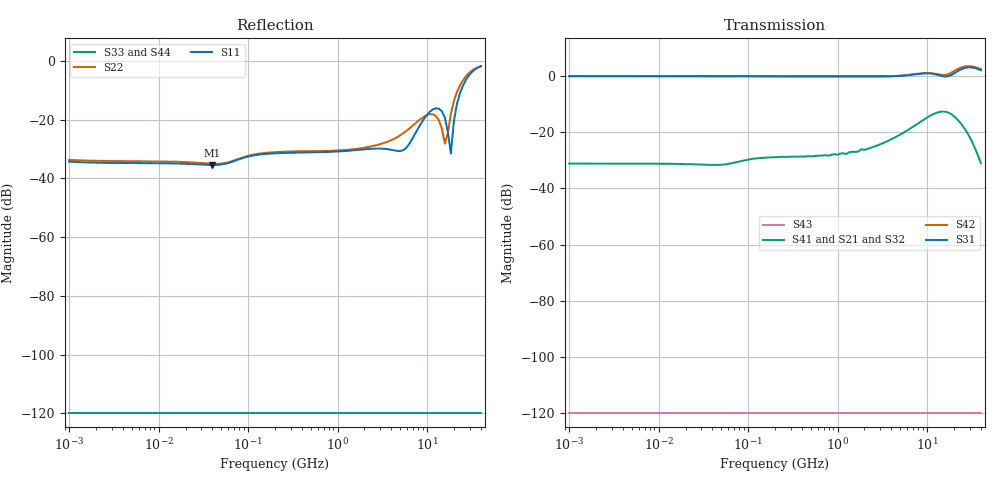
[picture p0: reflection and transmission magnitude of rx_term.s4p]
! Copyright 2015, Texas Instruments Incorporated. All rights reserved.
! Generated by program util_convert_s2p_term_to_s4p on 12-09-2015 11:37:60
!  1 ----xxxxxxxxxxxxxxxxxx---- 3
!  xxxxxxxxxxxxxxxxxx
! Termination looking in to RX ---> (Input) xxxxxxxxxxxxxxxxxx  (Output)
!  xxxxxxxxxxxxxxxxxx
!  2 ----xxxxxxxxxxxxxxxxxx---- 4
! FREQ  S11  S12  S13  S14
!  S21  S22  S23  S24
!  S31  S32  S33  S34
!  S41  S42  S43  S44
!  DB  ANG  DB  ANG  DB  ANG  DB  ANG
# HZ S DB R 50.00
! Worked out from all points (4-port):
!   139 points, 1 MHz to 40 GHz, reference 50 ohm
!   strongest paths, dB at 1 MHz, 13.59 MHz, 199.5 MHz, 2.929 GHz, 40 GHz:
!     S31: -0.2, -0.2, -0.2, -0.3, 1.9
!     S42: -0.2, -0.2, -0.2, -0.3, 2.4
!     S41: -31.2, -31.3, -29.0, -24.5, -31.0
!     S21: -31.2, -31.3, -29.0, -24.5, -31.0
!     S32: -31.2, -31.3, -29.0, -24.5, -31.0
!     S43: -120.0, -120.0, -120.0, -120.0, -120.0
!   lowest |S11| = -35.4 dB at 39.81 MHz (marker M1), VSWR 1.03, Z = 48.4 - j0.242 ohm
!   |S11| at or under -10 dB: start of sweep to 24.05 GHz
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1000000  -34.26 -160.3  -31.23 -178.5  -120.00 0.0  -120.00 0.0
         -31.24 -178.4  -33.66 -161.7  -120.00 0.0  -120.00 0.0
         -0.16 -0.4  -31.23 -178.5  -120.00 0.0  -120.00 0.0
         -31.24 -178.4  -0.17 -0.4  -120.00 0.0  -120.00 0.0
3.98107e7  -35.42 -171.5  -31.89 -175.4  -120.00 0.0  -120.00 0.0
           -31.72 -174.6  -34.99 -173.9  -120.00 0.0  -120.00 0.0
           -0.15 -0.1  -31.89 -175.4  -120.00 0.0  -120.00 0.0
           -31.72 -174.6  -0.16 -0.1  -120.00 0.0  -120.00 0.0
5.01187e9  -30.67 107.4  -20.90 174.9  -120.00 0.0  -120.00 0.0
           -20.93 174.8  -25.34 90.6  -120.00 0.0  -120.00 0.0
           -0.07 1.6  -20.90 174.9  -120.00 0.0  -120.00 0.0
           -20.93 174.8  0.01 3.1  -120.00 0.0  -120.00 0.0
1.25893e10  -16.09 -74.1  -13.20 72.3  -120.00 0.0  -120.00 0.0
            -13.25 72.3  -18.77 -52.0  -120.00 0.0  -120.00 0.0
            0.45 -8.2  -13.20 72.3  -120.00 0.0  -120.00 0.0
            -13.25 72.3  0.63 -4.8  -120.00 0.0  -120.00 0.0
1.84785e10  -31.53 -42.2  -13.52 -15.7  -120.00 0.0  -120.00 0.0
            -13.58 -15.5  -18.00 17.4  -120.00 0.0  -120.00 0.0
            0.17 -1.0  -13.52 -15.7  -120.00 0.0  -120.00 0.0
            -13.58 -15.5  0.99 1.9  -120.00 0.0  -120.00 0.0
2.32631e10  -11.12 -20.1  -16.53 -72.6  -120.00 0.0  -120.00 0.0
            -16.58 -72.3  -8.43 -14.8  -120.00 0.0  -120.00 0.0
            2.04 -4.3  -16.53 -72.6  -120.00 0.0  -120.00 0.0
            -16.58 -72.3  2.73 -4.1  -120.00 0.0  -120.00 0.0
4e10  -1.80 -93.5  -31.02 153.3  -120.00 0.0  -120.00 0.0
      -31.01 153.7  -1.77 -88.1  -120.00 0.0  -120.00 0.0
      1.94 -40.5  -31.02 153.3  -120.00 0.0  -120.00 0.0
      -31.01 153.7  2.35 -38.5  -120.00 0.0  -120.00 0.0
